(* 	
	Program Name: 	ACS_SAMPLE_BACK_AND_FORTH
	Purpose:		Example of a program that cycles motion back and forth
	When Executed:	Monitors current position, determines if extended or retracted, and executes a new move based on its current position and motion complete status
*)
PROGRAM ACS_SAMPLE_BACK_AND_FORTH
VAR_IN_OUT 
	Axis:ACS_DRIVE_TYPE;
END_VAR

VAR_INPUT
	ExtendPosition:REAL;
	RetractPosition:REAL;
	ProfileVelocity:REAL;
	ProfileAccelDecel:REAL;
	ProfileForce:REAL;	
END_VAR

VAR
	_readyToRumble:BOOL;
	_extended:BOOL;
	_midpoint:REAL;
END_VAR

(* 
	This program contains both the input and output scan and is intented to be a stand alone application
	Remember : The input scan should be one of the first things done in the program.  Then the processing.  
	Then the Output Scan.
	|->Input Scan
	|
	|->Processing (User Code)
	|
	|->Output Scan
*)

//Input Scan Routine
ACS_DRIVE_INPUT_SCAN(Axis:=Axis);

//Processing (User Code)

//Step 1. Initialize the drive
ACS_INITIALIZATION_NOBRAKE(Axis:=Axis);

//Step 2. Monitor Extended Status
_midpoint := (ExtendPosition - RetractPosition) / 2;
_extended := (Axis.InputCurrentPosition >= _midpoint);

//Step 3. Determine if we are Ready To Rumble (motion is possible)
_readyToRumble := (Axis.InputStatusDriveEnabled AND Axis.InputStatusDriveHomed AND NOT Axis.InputFaultActive);	

//Step 4. Run program based on extend or retracted state
IF _readyToRumble THEN
	
	IF _extended THEN
		ACS_MOVE_ABSOLUTE(Axis:=Axis,
			ProfilePosition:=RetractPosition,
			ProfileVelocity:=ProfileVelocity,
			ProfileAcceleration:=ProfileAccelDecel,
			ProfileDeceleration:=ProfileAccelDecel,
			ProfileForce:=ProfileForce);
			IF Axis.InputStatusDriveInMotion THEN
				ACS_CMD_CLEAR_START_MOTION(Axis:=Axis);
			ELSE
					ACS_CMD_START_MOTION(Axis:=Axis);
			END_IF
	ELSE
		ACS_MOVE_ABSOLUTE(Axis:=Axis,
			ProfilePosition:=ExtendPosition,
			ProfileVelocity:=ProfileVelocity,
			ProfileAcceleration:=ProfileAccelDecel,
			ProfileDeceleration:=ProfileAccelDecel,
			ProfileForce:=ProfileForce);
			IF Axis.InputStatusDriveInMotion THEN
				ACS_CMD_CLEAR_START_MOTION(Axis:=Axis);
			ELSE
					ACS_CMD_START_MOTION(Axis:=Axis);
			END_IF		
	END_IF

END_IF



//End processing (User Code)

//Output Scan Routine
ACS_DRIVE_OUTPUT_SCAN(Axis:=Axis);

END_PROGRAM
